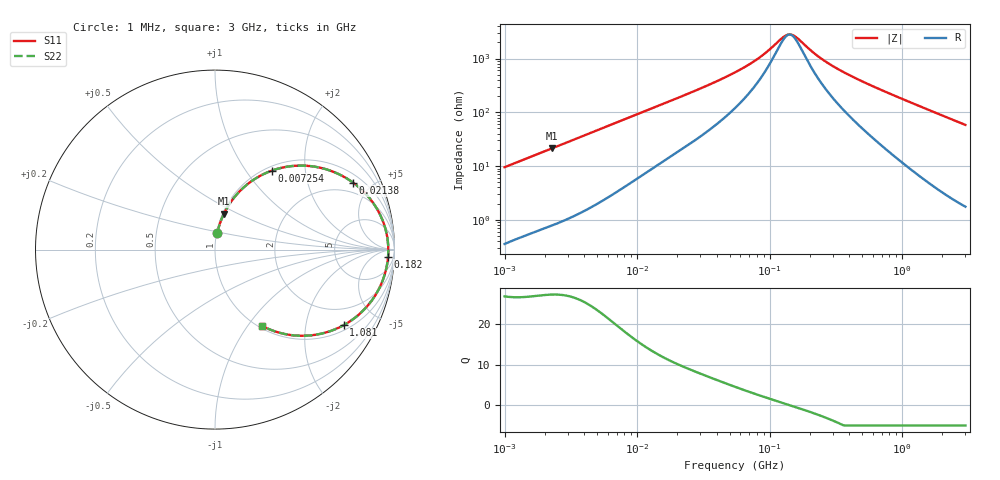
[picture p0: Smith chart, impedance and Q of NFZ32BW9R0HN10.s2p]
! NFZ32BW9R0HN10
# Hz S RI R 50
!Freq.(Hz) S11(Real) S11(Imag) S21(Real) S21(Imag) S12(Real) S12(Imag) S22(Real) S22(Imag)
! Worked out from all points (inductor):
!   401 points, 1 MHz to 3 GHz, reference 50 ohm
!   read as one part in series: L = 1.51 uH near 1.041 MHz
!   highest Q = 27.2 at 2.272 MHz (marker M1), where L = 1.49 uH
!   self-resonance near 141.4 MHz
!   S11 on the Smith chart (normalised r, x): 1 MHz: 1.01, +0.19; 7.254 MHz: 1.07, +1.34; 21.38 MHz: 1.40, +3.89; 182 MHz: 25, -28; 1.081 GHz: 1.20, -3.27; 3 GHz: 1.04, -1.17
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1000000  0.0124 0.0937  0.9876 -0.0937  0.9876 -0.0937  0.0124 0.0937
2271982  0.05 0.2003  0.95 -0.2003  0.95 -0.2003  0.05 0.2003
3823119  0.1214 0.3077  0.8786 -0.3077  0.8786 -0.3077  0.1214 0.3077
5266264  0.2026 0.3806  0.7974 -0.3806  0.7974 -0.3806  0.2026 0.3806
7254166  0.3185 0.4406  0.6815 -0.4406  0.6815 -0.4406  0.3185 0.4406
1.019448e7  0.4697 0.468  0.5303 -0.468  0.5303 -0.468  0.4697 0.468
1.461624e7  0.6313 0.4436  0.3687 -0.4436  0.3687 -0.4436  0.6313 0.4436
2.137957e7  0.7701 0.3724  0.2299 -0.3724  0.2299 -0.3724  0.7701 0.3724
3.320783e7  0.8748 0.2686  0.1252 -0.2686  0.1252 -0.2686  0.8748 0.2686
5.477226e7  0.9354 0.1588  0.0646 -0.1588  0.0646 -0.1588  0.9354 0.1588
8.338914e7  0.9574 0.0824  0.0426 -0.0824  0.0426 -0.0824  0.9574 0.0824
1.348146e8  0.9655 0.00716  0.0345 -0.00716  0.0345 -0.00716  0.9655 0.00716
1.520175e8  0.9656 -0.011  0.0344 0.011  0.0344 0.011  0.9656 -0.011
1.820241e8  0.9643 -0.0385  0.0357 0.0385  0.0357 0.0385  0.9643 -0.0385
2.094008e8  0.9621 -0.0607  0.0379 0.0607  0.0379 0.0607  0.9621 -0.0607
2.662515e8  0.9553 -0.1011  0.0447 0.1011  0.0447 0.1011  0.9553 -0.1011
3.594878e8  0.9394 -0.158  0.0606 0.158  0.0606 0.158  0.9394 -0.158
5.583748e8  0.8912 -0.2577  0.1088 0.2577  0.1088 0.2577  0.8912 -0.2577
8.005644e8  0.8152 -0.3497  0.1848 0.3497  0.1848 0.3497  0.8152 -0.3497
1.080907e9  0.7171 -0.421  0.2829 0.421  0.2829 0.421  0.7171 -0.421
1.782824e9  0.4924 -0.4803  0.5076 0.4803  0.5076 0.4803  0.4924 -0.4803
3e9  0.2598 -0.4237  0.7402 0.4237  0.7402 0.4237  0.2598 -0.4237
